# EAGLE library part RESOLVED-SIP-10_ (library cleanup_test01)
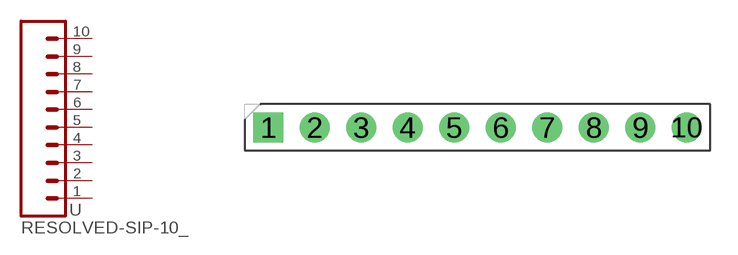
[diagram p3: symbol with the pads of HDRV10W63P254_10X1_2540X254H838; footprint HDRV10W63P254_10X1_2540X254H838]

Designator prefix -

## RESOLVED-SIP-10_2.54-SPACE-VERTICAL  [HDRV10W63P254_10X1_2540X254H838]
1  1  pas
2  2  pas
3  3  pas
4  4  pas
5  5  pas
6  6  pas
7  7  pas
8  8  pas
9  9  pas
10  10  pas

## Footprint HDRV10W63P254_10X1_2540X254H838 (pad centres in mm)
drill 1.1 pad 1.65 square: 1 0,0
drill 1.1 pad 1.65: 2 2.54,0; 3 5.08,0; 4 7.62,0; 5 10.16,0; 6 12.7,0; 7 15.24,0; 8 17.78,0; 9 20.32,0; 10 22.86,0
